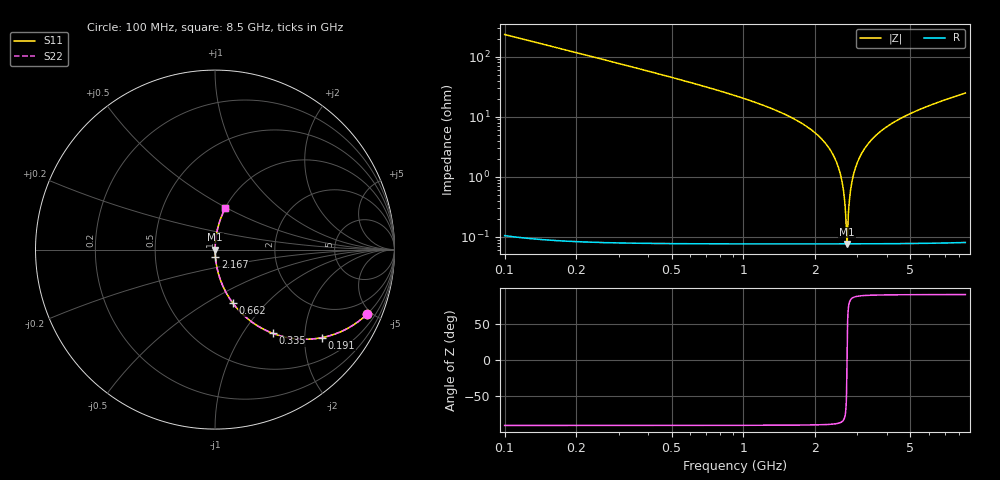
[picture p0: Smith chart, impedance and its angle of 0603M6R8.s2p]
! Created Wed Apr 18 16:07:22 2012
# hz S ma R 50
! 2 Port Network Data from SP1.SP block
! freq  magS11  angS11  magS21  angS21  magS12  angS12  magS22  angS22
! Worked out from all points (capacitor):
!   8401 points, 100 MHz to 8.5 GHz, reference 50 ohm
!   read as one part in series: C = 6.8 pF near 142 MHz
!   lowest |Z| = 76.6 mohm at 2.715 GHz (marker M1)
!   series resonance near 2.715 GHz, so ESL is about 510 pH
!   S11 on the Smith chart (normalised r, x): 100 MHz: 1.00, -4.67; 191 MHz: 1.00, -2.44; 335 MHz: 1.00, -1.38; 662 MHz: 1.00, -0.67; 2.167 GHz: 1.00, -0.08; 8.5 GHz: 1.00, +0.50
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1e8  0.9192 -23.2  0.3933 66.8  0.3933 66.8  0.9192 -23.2
1.91e8  0.773 -39.3  0.6339 50.6  0.6339 50.6  0.773 -39.3
3.35e8  0.5665 -55.4  0.8234 34.5  0.8234 34.5  0.5665 -55.4
6.62e8  0.3154 -71.5  0.9482 18.4  0.9482 18.4  0.3154 -71.5
1.5e9  0.1077 -83.4  0.9934 6.2  0.9934 6.2  0.1077 -83.4
2.167e9  0.03918 -86.6  0.9985 2.2  0.9985 2.2  0.03918 -86.6
2.388e9  0.02219 -86.8  0.999 1.3  0.999 1.3  0.02219 -86.8
2.538e9  0.01165 -85.6  0.9992 0.7  0.9992 0.7  0.01165 -85.6
2.622e9  0.006044 -82.4  0.9992 0.3  0.9992 0.3  0.006044 -82.4
2.651e9  0.004167 -79.2  0.9992 0.2  0.9992 0.2  0.004167 -79.2
2.689e9  0.001809 -64.9  0.9992 0.1  0.9992 0.1  0.001809 -64.9
2.715e9  0.0007654 1.7  0.9992 -0.0  0.9992 -0.0  0.0007654 1.7
2.741e9  0.001835 65.3  0.9992 -0.1  0.9992 -0.1  0.001835 65.3
2.778e9  0.004056 78.9  0.9992 -0.2  0.9992 -0.2  0.004056 78.9
2.809e9  0.00595 82.3  0.9992 -0.3  0.9992 -0.3  0.00595 82.3
2.9e9  0.01144 85.5  0.9992 -0.7  0.9992 -0.7  0.01144 85.5
3.083e9  0.02205 86.7  0.999 -1.3  0.999 -1.3  0.02205 86.7
3.361e9  0.03717 86.7  0.9985 -2.1  0.9985 -2.1  0.03717 86.7
4.3e9  0.08221 84.7  0.9958 -4.7  0.9958 -4.7  0.08221 84.7
5.7e9  0.1397 81.7  0.9894 -8.0  0.9894 -8.0  0.1397 81.7
7.1e9  0.1915 78.7  0.9807 -11.0  0.9807 -11.0  0.1915 78.7
8.5e9  0.2402 75.9  0.9699 -13.9  0.9699 -13.9  0.2402 75.9
